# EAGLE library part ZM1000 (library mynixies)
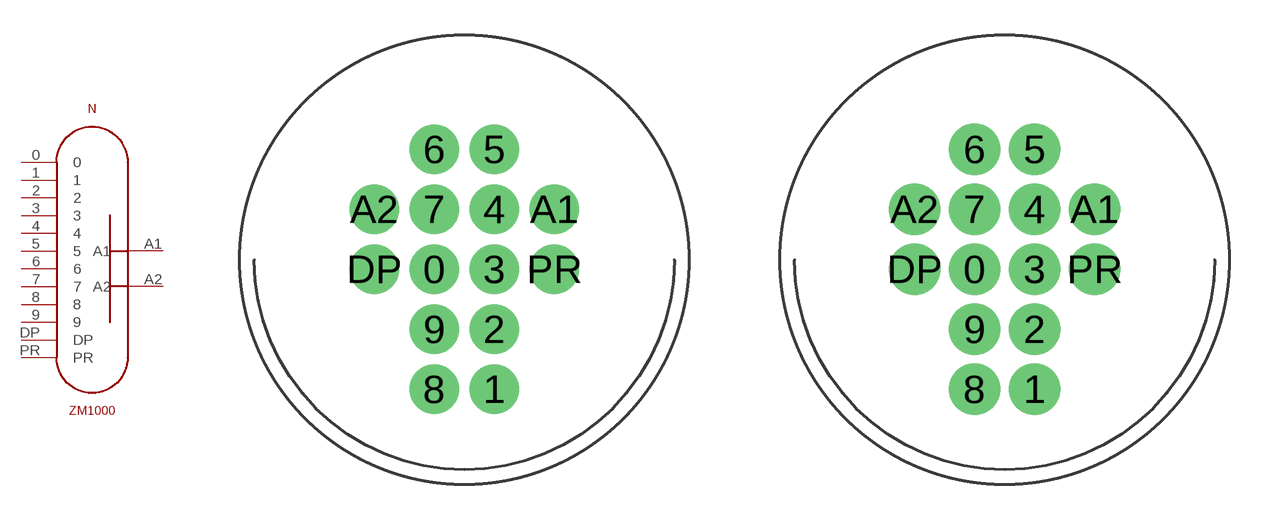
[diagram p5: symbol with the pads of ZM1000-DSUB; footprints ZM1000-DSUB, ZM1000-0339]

Designator prefix N

## ZM1000D-SUB  [ZM1000-DSUB]
0  0  pas
1  1  pas
2  2  pas
3  3  pas
4  4  pas
5  5  pas
6  6  pas
7  7  pas
8  8  pas
9  9  pas
A1  A1  pas
A2  A2  pas
DP  DP  pas
PR  PR  pas

## ZM1000  [ZM1000-0339]
Pads as for ZM1000-DSUB

## Footprint ZM1000-DSUB (pad centres in mm)
drill 1.4: 0 -1.27,-0.4; 1 1.27,-5.48; 2 1.27,-2.94; 3 1.27,-0.4; 4 1.27,2.14; 5 1.27,4.68; 6 -1.27,4.68; 7 -1.27,2.14; 8 -1.27,-5.48; 9 -1.27,-2.94; A1 3.81,2.14; A2 -3.81,2.14; DP -3.81,-0.4; PR 3.81,-0.4

## Footprint ZM1000-0339 (pad centres in mm)
drill 1.45: 0 -1.27,-0.4; 1 1.27,-5.48; 2 1.27,-2.94; 3 1.27,-0.4; 4 1.27,2.14; 5 1.27,4.68; 6 -1.27,4.68; 7 -1.27,2.14; 8 -1.27,-5.48; 9 -1.27,-2.94; A1 3.81,2.14; A2 -3.81,2.14; DP -3.81,-0.4; PR 3.81,-0.4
